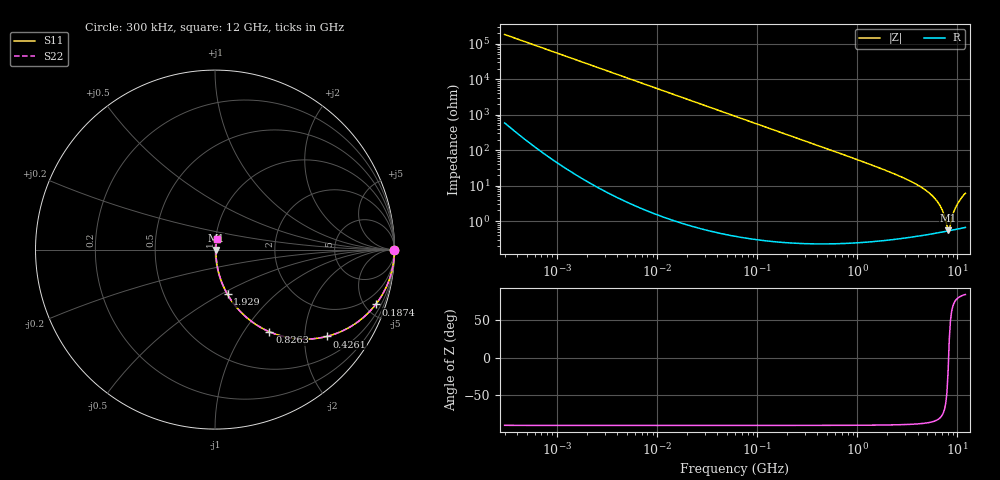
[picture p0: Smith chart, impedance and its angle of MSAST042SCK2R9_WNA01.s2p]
! MSAST042SCK2R9_WNA01  S-PARAMETER MODEL  ( General Type )
! Model Generated by TAIYO YUDEN Corporation (http://www.ty-top.com)
! Version 1.0
! TAIYO YUDEN Control No. 150820
! Copyright(c) 2015 TAIYO YUDEN CO.,LTD. All Rights Reserved.
! Product Description (link to TY-COMPAS)
! https://ds.yuden.co.jp/TYCOMPAS/or/detail?pn=MSAST042SCK2R9AWNA01&u=M
! Products Name : Multilayer Ceramic Capacitors
! Characteristics :
!  Capacitance : 2.9 pF , Rated Voltage : 25V , TCC : CK / C0K
!  Case Size : 0.4 x 0.2 / 0.016 x 0.008 [mm/inch] , Thickness : 0.2 / 0.008 [mm/inch]
!  (Conditions: Temperature = 25 degC , DC Bias Current/Voltage = 0A / 0V)
! External Node Assignments :
!  1  o---| |---o  2
! GND o---------o GND
! Frequency Range : 0.3MHz  -  12000MHz  [ 401 STEP ]
# MHz S RI R 50
! Freq[MHz].  S11 Real  S11 Imag  S21 Real  S21 Imag  S12 Real  S12 Imag  S22 Real  S22 Imag
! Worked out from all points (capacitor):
!   401 points, 300 kHz to 12 GHz, reference 50 ohm
!   read as one part in series: C = 2.9 pF near 316.3 kHz
!   lowest |Z| = 557 mohm at 8.065 GHz (marker M1)
!   series resonance near 8.156 GHz, so ESL is about 130 pH
!   S11 on the Smith chart (normalised r, x): 300 kHz: open; 187.4 MHz: 1.00, -5.86; 426.1 MHz: 1.00, -2.57; 826.3 MHz: 1.00, -1.32; 1.929 GHz: 1.01, -0.54; 12 GHz: 1.01, +0.12
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0.3  1 -0.000546  2.06e-06 0.000546  2.06e-06 0.000546  1 -0.000546
1.769972  1 -0.00322  1.21e-05 0.00322  1.21e-05 0.00322  1 -0.00322
10.44266  0.9996 -0.019  0.000367 0.019  0.000367 0.019  0.9996 -0.019
60  0.9882 -0.108  0.0118 0.108  0.0118 0.108  0.9882 -0.108
187.4445  0.8953 -0.3057  0.1047 0.3057  0.1047 0.3057  0.8953 -0.3057
353.9943  0.7054 -0.4551  0.2946 0.4551  0.2946 0.4551  0.7054 -0.4551
426.1204  0.6227 -0.4838  0.3773 0.4838  0.3773 0.4838  0.6227 -0.4838
826.3444  0.3026 -0.4576  0.6974 0.4576  0.6974 0.4576  0.3026 -0.4576
1229.528  0.1615 -0.3651  0.8385 0.3651  0.8385 0.3651  0.1615 -0.3651
1928.972  0.0697 -0.2494  0.9303 0.2494  0.9303 0.2494  0.0697 -0.2494
2088.533  0.0594 -0.2305  0.9406 0.2305  0.9406 0.2305  0.0594 -0.2305
3740.715  0.0168 -0.1137  0.9832 0.1137  0.9832 0.1137  0.0168 -0.1137
5420.343  0.00748 -0.0561  0.9925 0.0561  0.9925 0.0561  0.00748 -0.0561
6699.894  0.0055 -0.0266  0.9945 0.0266  0.9945 0.0266  0.0055 -0.0266
7254.098  0.00524 -0.0159  0.9948 0.0159  0.9948 0.0159  0.00524 -0.0159
7854.144  0.00523 -0.00529  0.9948 0.00529  0.9948 0.00529  0.00523 -0.00529
8064.993  0.00528 -0.00169  0.9947 0.00169  0.9947 0.00169  0.00528 -0.00169
8503.825  0.00547 0.00609  0.9945 -0.00609  0.9945 -0.00609  0.00547 0.00609
9207.246  0.00598 0.0175  0.994 -0.0175  0.994 -0.0175  0.00598 0.0175
9968.853  0.00679 0.029  0.9932 -0.029  0.9932 -0.029  0.00679 0.029
11083.22  0.00844 0.0459  0.9916 -0.0459  0.9916 -0.0459  0.00844 0.0459
12000  0.0102 0.0597  0.9898 -0.0597  0.9898 -0.0597  0.0102 0.0597
